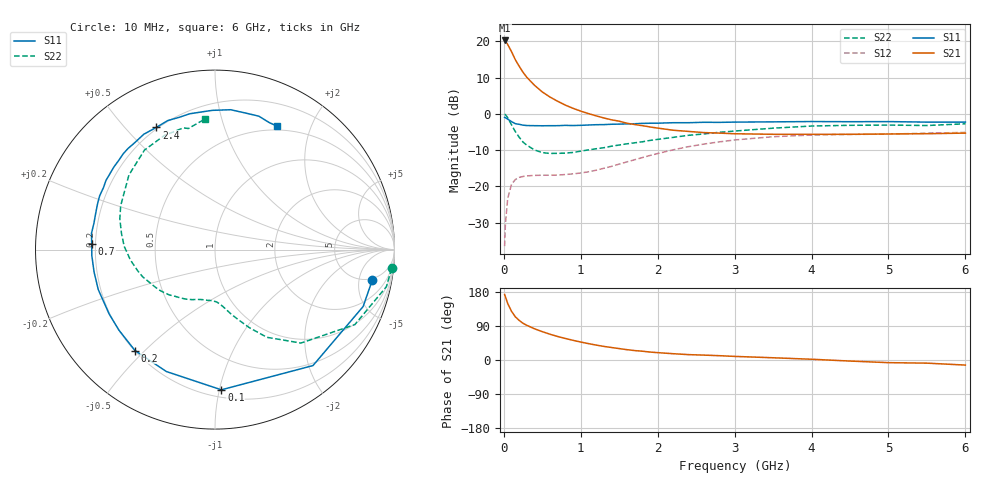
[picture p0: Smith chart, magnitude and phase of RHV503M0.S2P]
! SIEMENS Small Signal Semiconductors
! BFR106
! Si NPN RF Bipolar Junction Transistor in SOT23
! VCE = 0.5 V  IC = 3 mA
! Common Emitter S-Parameters:  August  1996
# GHz  S  MA  R  50
!  f  S11  S21  S12  S22
! GHz  MAG  ANG  MAG  ANG  MAG  ANG  MAG  ANG
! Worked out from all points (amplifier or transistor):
!   36 points, 10 MHz to 6 GHz, reference 50 ohm
!   highest |S21| = 20.2 dB at 10 MHz (marker M1)
!   |S21| within 3 dB of that: start of sweep to 97.51 MHz
!   unconditionally stable (mu >= 1): 664.5 MHz to end of sweep
!   at 250 MHz: K = 0.42, MSG = 14.4 dB, |S12| = -17.3 dB
!   at 1.4 GHz: K = 1.31, MAG = 3.1 dB, |S12| = -14.5 dB
!   at 6 GHz: K = 1.03, MAG = -1.1 dB, |S12| = -5.1 dB
!   S11 on the Smith chart (normalised r, x): 10 MHz: 4.70, -7.78; 100 MHz: 0.25, -1.01; 200 MHz: 0.20, -0.47; 700 MHz: 0.19, +0.02; 2.4 GHz: 0.19, +0.61; 6 GHz: 0.46, +1.53
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0.01  0.8932 -10.8  10.28 172.8  0.015 85.9  0.9896 -6.1
0.02  0.8842 -21.0  10.08 167.2  0.0298 78.5  0.977 -12.2
0.05  0.8459 -49.8  9.058 149.2  0.0679 63.2  0.8841 -28.2
0.1  0.782 -87.4  7.196 128.4  0.1069 45.7  0.7073 -47.4
0.15  0.7314 -111.7  5.563 113.8  0.1245 34.9  0.5677 -59.4
0.2  0.7176 -128.4  4.527 104.4  0.1332 29.0  0.4759 -66.2
0.25  0.6985 -140.0  3.739 96.8  0.1371 25.1  0.4075 -72.0
0.3  0.6903 -148.7  3.183 91.4  0.1396 23.3  0.3692 -76.1
0.4  0.6875 -161.1  2.47 82.3  0.1419 21.1  0.3179 -82.4
0.5  0.6852 -169.5  2.006 74.8  0.1426 21.0  0.2923 -87.9
0.6  0.6872 -177.2  1.706 68.0  0.1426 22.1  0.2847 -93.4
0.7  0.6877 177.3  1.49 62.0  0.1434 23.9  0.2857 -99.0
0.9  0.6903 167.7  1.192 51.9  0.149 29.2  0.2938 -109.2
1.1  0.7022 158.8  1.009 43.2  0.1591 35.4  0.3189 -120.0
1.6  0.7276 140.7  0.743 27.3  0.2177 45.2  0.3865 -145.0
2.2  0.7553 121.7  0.595 16.6  0.3191 42.9  0.4741 -172.8
2.4  0.7553 115.7  0.573 14.2  0.3533 39.9  0.5062 178.0
3.5  0.7759 91.2  0.523 5.9  0.4842 20.1  0.635 139.0
4.5  0.7796 77.2  0.523 -2.8  0.5205 4.2  0.6955 114.0
5  0.7825 71.8  0.528 -7.0  0.5262 -1.8  0.7008 104.6
5.5  0.7697 67.0  0.533 -8.3  0.5417 -4.6  0.6908 102.4
6  0.7696 63.1  0.543 -13.4  0.5555 -11.1  0.7301 94.3
